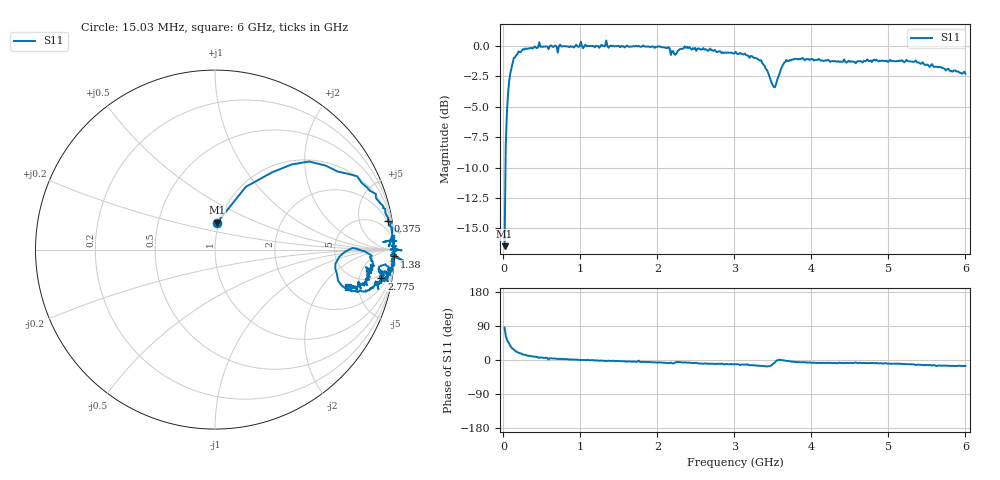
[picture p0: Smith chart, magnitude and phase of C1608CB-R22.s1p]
!	Network	Analyzer	HP8753E.07.74:	Oct	30	2002	Serial	No.	JP38451487
!	Hewlett-Packard
!	7	Sep	2009	10:04:20
!	Frequency	S11
#	HZ	S	RI	R	50
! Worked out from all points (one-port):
!   400 points, 15.03 MHz to 6 GHz, reference 50 ohm
!   lowest |S11| = -16.5 dB at 15.03 MHz (marker M1), VSWR 1.35, Z = 48.9 + j15 ohm
!   |S11| at or under -10 dB: start of sweep to 26.73 MHz
!   S11 on the Smith chart (normalised r, x): 15.03 MHz: 0.98, +0.30; 375 MHz: 2, +12; 1.38 GHz: 3, -52; 2.775 GHz: 4, -10; 6 GHz: 3.69, -3.73
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1.502992e7  0.0119 0.15
3.002985e7  0.172 0.35
7.502962e7  0.524 0.491
1.350293e8  0.793 0.408
1.95029e8  0.896 0.31
3.750281e8  0.962 0.16
4.650277e8  1.03 0.093
5.550272e8  0.989 0.109
5.850271e8  0.969 0.0185
6.00027e8  0.992 0.08
7.050265e8  0.936 0.042
7.650262e8  0.991 0.0565
1.335023e9  1.05 -0.0624
1.380023e9  0.997 -0.0383
1.515022e9  0.985 -0.0512
1.755021e9  1 -0.0274
1.785021e9  0.986 -0.0958
2.205019e9  0.937 -0.152
2.265019e9  0.95 -0.0821
2.775016e9  0.927 -0.161
3.015015e9  0.927 -0.186
3.420013e9  0.763 -0.233
3.510012e9  0.67 -0.105
3.585012e9  0.766 0.00931
3.765011e9  0.876 -0.0642
4.515007e9  0.856 -0.115
5.265004e9  0.848 -0.167
6e9  0.739 -0.208
